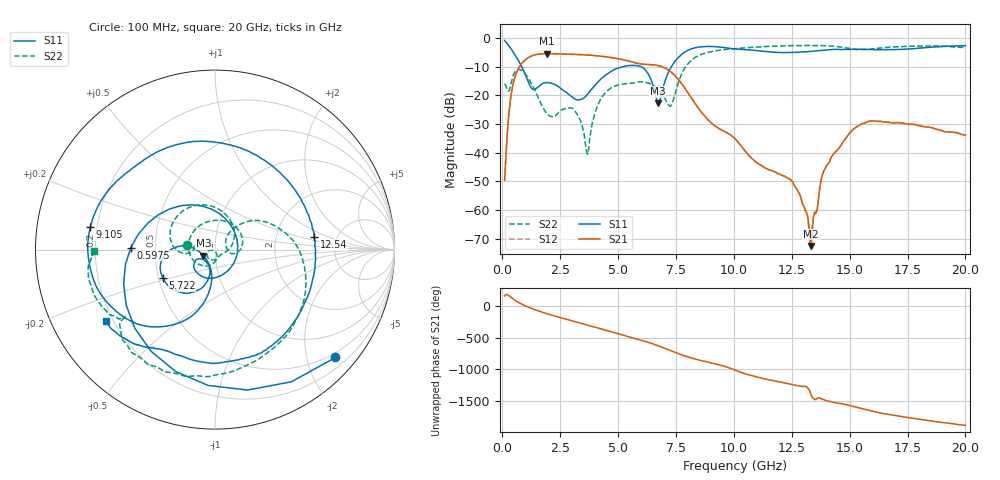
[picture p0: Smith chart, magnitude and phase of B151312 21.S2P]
!  2-Port S-parameters saved by WinCal
! VAR MeasName=S-Parameters (CALIBRATED_DATA) read from VNA (N5244A)
! VAR MeasDate=12/8/2015 5:45:04 PM
! VAR NAME=B151312 21
! VAR FILENAME=B151312 21.S2P
! VAR DATE=12/8/2015 5:45:04 PM
! VAR PHYS_PORTS=1,2
# Hz S DB R 50
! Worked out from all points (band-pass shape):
!   401 points, 100 MHz to 20 GHz, reference 50 ohm
!   highest |S21| = -5.53 dB at 1.941 GHz (marker M1); lowest = -72.6 dB at 13.33 GHz (marker M2)
!   |S21| within 3 dB of the highest: 884.8 MHz to 5.664 GHz (4.779 GHz wide, 146 % of centre)
!   lowest |S11| = -22.8 dB at 6.717 GHz (marker M3), VSWR 1.16, Z = 43.9 - j2.95 ohm
!   |S11| at or under -10 dB: 836.4 MHz to 5.238 GHz (4.402 GHz wide, 145 % of centre); 5.981 GHz to 7.307 GHz (1.326 GHz wide, 20 % of centre)
!   |S22| runs from -40.6 to -2.6 dB; largest |S21 - S12| = 0.0017
!   S11 on the Smith chart (normalised r, x): 100 MHz: 0.40, -2.56; 597.5 MHz: 0.36, +0.01; 5.722 GHz: 0.53, -0.19; 9.105 GHz: 0.17, +0.09; 12.54 GHz: 3.35, +0.69; 20 GHz: 0.17, -0.29
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1e8  -0.91 -41.9  -49.66 158.2  -49.94 159.4  -15.96 170.5
3.4875e8  -3.49 -122.2  -21.80 144.2  -21.78 144.1  -17.05 -172.3
5.975e8  -6.58 178.7  -12.46 77.6  -12.46 77.6  -11.34 156.9
1.14475e9  -15.81 57.0  -6.79 -21.0  -6.79 -21.0  -14.33 66.2
1.94075e9  -15.58 -116.1  -5.53 -123.3  -5.53 -123.3  -26.47 -31.0
2.5875e9  -18.02 -150.2  -5.64 168.8  -5.64 168.7  -25.08 -88.0
3.43325e9  -21.36 -121.6  -5.87 84.0  -5.86 84.0  -30.06 -172.7
3.682e9  -19.66 -107.2  -5.97 59.1  -5.96 59.0  -40.59 -109.2
4.32875e9  -13.83 -105.9  -6.44 -6.8  -6.44 -6.8  -20.41 -110.3
5.72175e9  -9.62 -151.7  -8.67 -152.3  -8.65 -152.3  -15.70 82.1
6.71675e9  -22.80 -152.6  -9.65 95.0  -9.66 94.9  -18.07 -6.5
6.7665e9  -22.79 -132.5  -9.74 88.2  -9.75 88.2  -18.48 -9.0
7.264e9  -10.58 -101.5  -11.78 17.8  -11.76 17.7  -23.87 18.8
7.861e9  -5.05 -129.7  -17.29 -65.0  -17.25 -65.3  -10.80 34.4
9.10475e9  -3.02 169.8  -30.20 177.3  -30.25 176.9  -4.67 -35.7
1.005e10  -3.86 132.1  -35.16 69.4  -35.21 69.0  -3.76 -65.0
1.25375e10  -5.10 7.3  -50.20 -161.6  -50.24 -161.4  -2.68 -111.6
1.33335e10  -4.71 -29.9  -72.57 37.9  -71.08 33.0  -2.67 -122.4
1.338325e10  -4.69 -32.0  -67.93 3.8  -66.34 14.5  -2.68 -123.0
1.427875e10  -4.05 -64.5  -40.89 -76.2  -40.79 -75.7  -2.87 -136.3
1.67165e10  -4.12 -112.6  -29.55 88.9  -29.40 88.9  -3.24 -148.2
2e10  -2.79 -146.9  -33.90 -82.9  -33.96 -84.2  -3.40 -179.3
